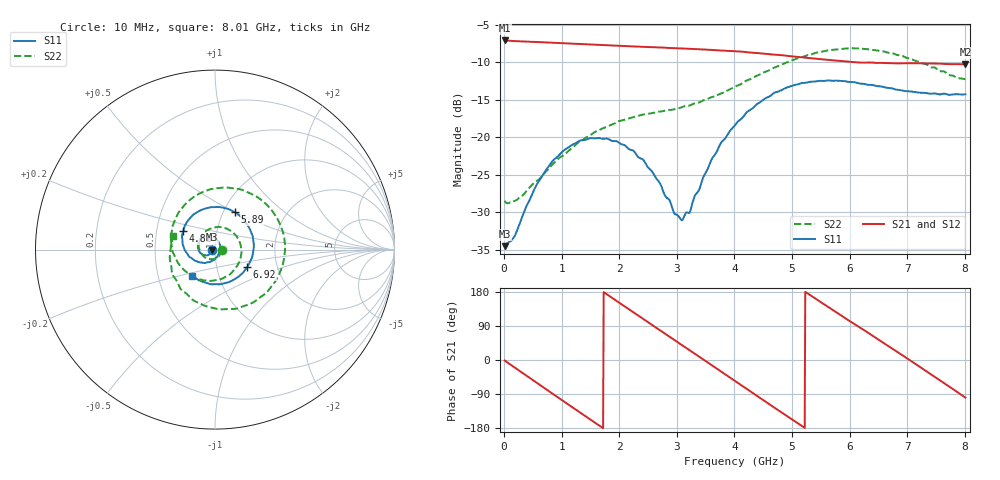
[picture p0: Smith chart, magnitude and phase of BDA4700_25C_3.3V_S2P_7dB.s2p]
!Agilent Technologies,E5071B,MY42404982,A.09.10
!Date: Mon Oct 20 18:05:56 2025
!Data & Calibration Information:
!Freq	S11:SOLT2(ON)	S21:SOLT2(ON)	S12:SOLT2(ON)	S22:SOLT2(ON)
# Hz S RI R 50
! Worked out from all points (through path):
!   801 points, 10 MHz to 8.01 GHz, reference 50 ohm
!   highest |S21| = -7.11 dB at 10 MHz (marker M1); lowest = -10.3 dB at 8.01 GHz (marker M2)
!   group delay of S21, straight-line fit = 283 ps
!   lowest |S11| = -34.5 dB at 10 MHz (marker M3), VSWR 1.04, Z = 48.2 - j0.0877 ohm
!   |S11| at or under -10 dB: start of sweep to end of sweep
!   |S22| runs from -28.8 to -8.1 dB; largest |S21 - S12| = 0.0051
!   S11 on the Smith chart (normalised r, x): 10 MHz: 0.96, -0.00; 4.81 GHz: 0.69, +0.15; 5.89 GHz: 1.13, +0.50; 6.92 GHz: 1.40, -0.28; 8.01 GHz: 0.75, -0.23
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1e7  -0.0187 -0.00091  0.4408 -0.00949  0.4407 -0.00993  0.0376 -0.00291
1.7e8  -0.0192 -0.00945  0.4147 -0.1374  0.4144 -0.1372  0.0329 -0.0177
3.3e8  -0.0238 -0.0189  0.3547 -0.2503  0.3546 -0.2505  0.0236 -0.0336
7.1e8  -0.0491 -0.0322  0.1104 -0.4136  0.1104 -0.4137  -0.0217 -0.0538
1.02e9  -0.0772 -0.0225  -0.1262 -0.4037  -0.1261 -0.4038  -0.0673 -0.0334
1.35e9  -0.0949 0.00736  -0.3274 -0.2589  -0.3275 -0.2591  -0.0906 0.028
1.64e9  -0.0898 0.041  -0.4081 -0.0595  -0.4084 -0.0595  -0.0664 0.0887
1.93e9  -0.0658 0.0671  -0.3785 0.1506  -0.3786 0.1504  -0.00043 0.1238
2.32e9  -0.0197 0.0715  -0.1899 0.3534  -0.1899 0.3531  0.1014 0.0939
2.68e9  0.0177 0.0478  0.0598 0.3917  0.0592 0.3913  0.1473 -0.00541
3.1e9  0.0269 -0.00788  0.3068 0.2403  0.3049 0.242  0.0933 -0.1286
3.54e9  -0.0125 -0.0605  0.3798 -0.046  0.3797 -0.0465  -0.0516 -0.1725
4.01e9  -0.1002 -0.0662  0.2125 -0.3073  0.2129 -0.3067  -0.2016 -0.0799
4.4e9  -0.1667 -0.00581  -0.0347 -0.3619  -0.0342 -0.3624  -0.2445 0.0803
4.81e9  -0.1765 0.1039  -0.2597 -0.2373  -0.258 -0.2388  -0.1626 0.2563
5.35e9  -0.068 0.224  -0.3273 0.0717  -0.3275 0.07  0.109 0.3401
5.89e9  0.1094 0.2093  -0.1293 0.2938  -0.1296 0.2929  0.3564 0.1539
6.28e9  0.1958 0.1109  0.0757 0.3042  0.0798 0.302  0.3776 -0.0832
6.68e9  0.2108 -0.0241  0.2519 0.1826  0.2528 0.1818  0.2381 -0.277
6.92e9  0.1797 -0.0969  0.3036 0.0655  0.3034 0.0638  0.1062 -0.331
7.48e9  0.0293 -0.1932  0.2194 -0.2178  0.2195 -0.2185  -0.1927 -0.2178
8.01e9  -0.1273 -0.1453  -0.0494 -0.3012  -0.049 -0.3015  -0.2322 0.0733
